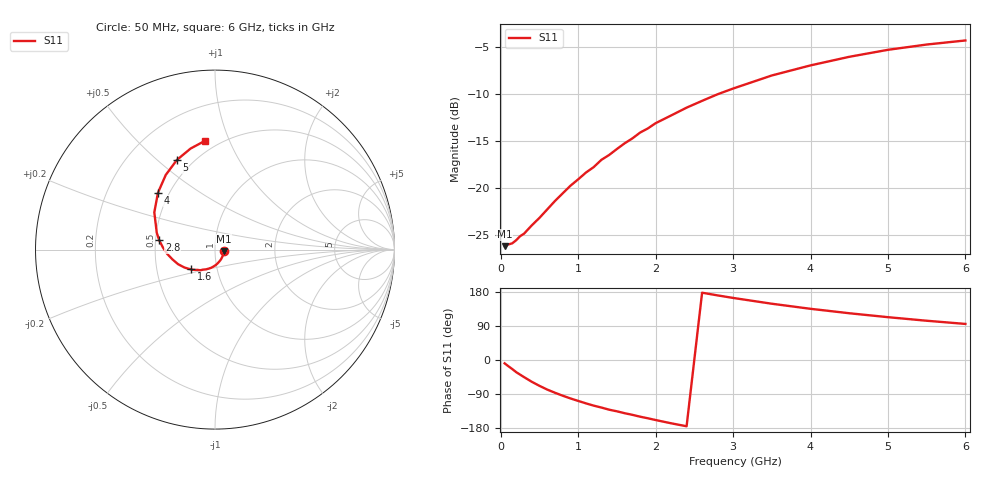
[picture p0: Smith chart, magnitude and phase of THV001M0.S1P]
! SIEMENS Discrete & RF Semiconductors
! BAS70
! Si Schottky Diode in SOT23
! IF = 1 mA
! S-Parameters:  February  1997
# GHz  S  MA  R  50
!  f  S11
! GHz  MAG  ANG
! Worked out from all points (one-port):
!   34 points, 50 MHz to 6 GHz, reference 50 ohm
!   lowest |S11| = -26.2 dB at 50 MHz (marker M1), VSWR 1.10, Z = 55.1 - j0.829 ohm
!   |S11| at or under -10 dB: start of sweep to 2.81 GHz
!   S11 on the Smith chart (normalised r, x): 50 MHz: 1.10, -0.02; 1.6 GHz: 0.75, -0.17; 2.8 GHz: 0.52, +0.06; 4 GHz: 0.43, +0.34; 5 GHz: 0.41, +0.58; 6 GHz: 0.42, +0.82
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0.05  0.04908 -8.8
0.15  0.05085 -24.1
0.2  0.05283 -32.1
0.25  0.05545 -38.6
0.3  0.05714 -45.0
0.5  0.0694 -68.2
0.7  0.08532 -86.4
0.8  0.09369 -94.2
0.9  0.1028 -101.4
1.1  0.1208 -114.4
1.2  0.1292 -120.4
1.3  0.1412 -125.5
1.4  0.1499 -131.1
1.6  0.1729 -140.4
1.7  0.1836 -144.7
1.8  0.1972 -149.6
1.9  0.2074 -153.8
2  0.2212 -158.4
2.2  0.243 -167.0
2.4  0.2675 -174.9
2.8  0.3151 170.5
3  0.3379 163.8
3.5  0.3966 148.5
4  0.4487 135.1
4.5  0.4984 123.4
5  0.543 113.0
5.5  0.5792 103.6
6  0.6089 95.2
